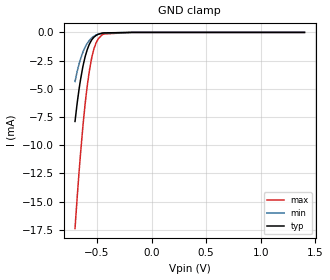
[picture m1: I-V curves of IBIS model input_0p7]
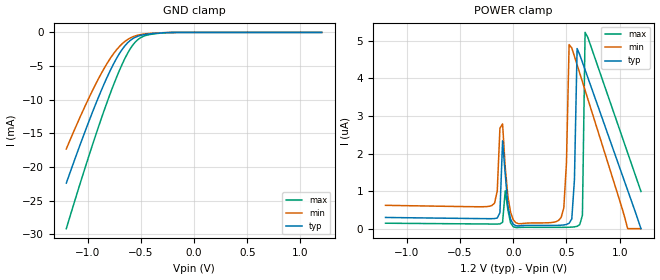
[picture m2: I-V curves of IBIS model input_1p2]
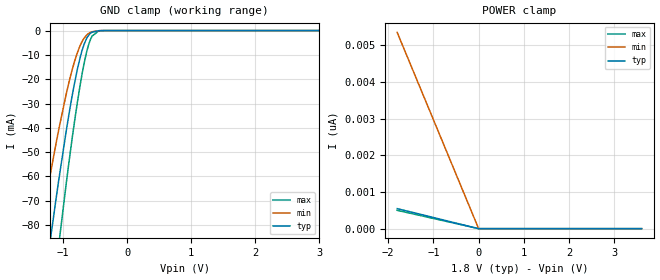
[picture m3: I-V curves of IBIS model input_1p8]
|Texas Instruments Incorporated
| 8-Bit Dual-Supply Bus Transceiver With Configurable Voltage Translation and
| 3-State Outputs
[IBIS Ver]   4.2
[File name]   sn74axc8t245.ibs
[Date]   03/06/2020
[File Rev]   1.2
[Source]
| Texas Instruments Incorporated.
| Analog-eLab Design Center, HPA
| 12500 TI Blvd
| Dallas, TX -75243
[Notes]
| Rev 1.2: 12/018/2023
| - Added input_1p2, 2p5, io_1p2 and io_2p5 model.
| Rev 1.1: 03/06/2020
| - Added input_1p8 and io_1p8 model.
| Rev 1.0: 06/08/2017
| - Initial version of the model
| - Model generated from simulations in SPECTRE
| - Model matched to SPICE simulation
| - C_comp although listed in numerical order of value are
|   obtained from varying PVT conditions. For PVT conditions for
|   each specific value refer the buffer description under
|   respective [Model]. IBIS model user is responsible for using
|   appropriate C_comp to simulate for Signal Integrity.
[Disclaimer]
| This model is designed as an aid for customers of Texas Instruments.
| TI and its licensors and suppliers make no warranties, either expressed
| or implied, with respect to this  model, including the warranties of
| merchantability or fitness for a particular purpose. The model is
| provided solely on an "as is" basis. The entire risk as to its quality
| and performance is with the customer.
[Copyright]
(C) Copyright 2017 Texas Instruments Incorporated.All rights reserved.
|   SN74AXC8T245PW
| Marketing part#   Digital Voltage Range   Package-type   #pins
| SN74AXC8T245PW   0.65V-3.6V   TSSOP   24
[Component]   SN74AXC8T245PW
[Manufacturer]  TI
[Package]   |24 TSSOP - PW package
|   typ   min   max
R_pkg   0.1143375   0.06811   0.12769
L_pkg   3.405334167nH   2.85598nH   4.17092nH
C_pkg   0.565412083pF   0.46044pF   0.71557pF
[Pin]  signal_name model_name   R_pin   L_pin   C_pin
1   VCCA   power   0.06958   3.86966nH   0.71557pF
2   DIR1   input   0.12094   3.80225nH   0.66679pF
3   A1   io   0.12769   3.54754nH   0.57242pF
4   A2   io   0.12362   3.25170nH   0.50771pF
5   A3   io   0.11601   3.02250nH   0.49462pF
6   A4   io   0.10931   2.86990nH   0.46105pF
7   A5   io   0.10845   2.85719nH   0.46044pF
8   A6   io   0.11376   2.99109nH   0.49241pF
9   A7   io   0.11998   3.20023nH   0.50408pF
10   A8   io   0.12312   3.48368nH   0.56447pF
11   DIR2   input   0.12091   3.81199nH   0.66374pF
12   GND   gnd   0.11675   4.13953nH   0.67876pF
13   GND   gnd   0.06811   3.82650nH   0.71298pF
14   B8   io   0.12091   3.81016nH   0.66711pF
15   B7   io   0.12766   3.55445nH   0.57259pF
16   B6   io   0.12359   3.25719nH   0.50787pF
17   B5   io   0.11599   3.02618nH   0.49474pF
18   B4   io   0.10929   2.87119nH   0.46118pF
19   B3   io   0.10845   2.85598nH   0.46051pF
20   B2   io   0.11377   2.98788nH   0.49236pF
21   B1   io   0.12   3.19513nH   0.50408pF
22   nOE   input   0.12314   3.47698nH   0.56494pF
23   VCCB   power   0.12375   3.84820nH   0.66804pF
24   VCCB   power   0.11932   4.17092nH   0.68143pF
|   SN74AXC8T245RHL
| Marketing part#   Digital Voltage Range   Package-type   #pins
| SN74AXC8T245RHL   0.65V-3.6V   YQFN   24
[Component]   SN74AXC8T245RHL
[Manufacturer]  TI
[Package]   |24 YQFN - RHL package
|   typ   min   max
R_pkg   0.085   0.058   0.116
L_pkg   1.593n   1.101n   2.229n
C_pkg   0.258p   0.219p   0.337p
[Pin]  signal_name model_name   R_pin   L_pin   C_pin
1   VCCA   power   0.0589   1.5334n   0.3373p
2   DIR1   input   0.1148   2.1925n   0.2676p
3   A1   io   0.0984   1.7889n   0.2917p
4   A2   io   0.0841   1.4994n   0.2570p
5   A3   io   0.0723   1.2607n   0.2333p
6   A4   io   0.0655   1.1245n   0.2200p
7   A5   io   0.0637   1.1101n   0.2185p
8   A6   io   0.0688   1.2432n   0.2289p
9   A7   io   0.0788   1.4543n   0.2506p
10   A8   io   0.0925   1.7374n   0.2753p
11   DIR2   input   0.1138   2.1938n   0.2623p
12   GND   gnd   0.1074   2.0415n   0.2530p
13   GND   gnd   0.0585   1.5096n   0.3326p
14   B8   io   0.1153   2.1253n   0.2676p
15   B7   io   0.0992   1.7605n   0.2916p
16   B6   io   0.0837   1.4781n   0.2571p
17   B5   io   0.0716   1.2733n   0.2332p
18   B4   io   0.0645   1.1262n   0.2200p
19   B3   io   0.0636   1.1010n   0.2188p
20   B2   io   0.0699   1.2254n   0.2290p
21   B1   io   0.0807   1.4310n   0.2511p
22   nOE   input   0.0943   1.7202n   0.2780p
23   VCCB   power   0.1164   2.2294n   0.2692p
24   VCCB   power   0.1093   2.0732n   0.2573p
|   SN74AXC8T245RJW
| Marketing part#   Digital Voltage Range   Package-type   #pins
| SN74AXC8T245RJW   0.65V-3.6V   uQFN   24
[Component]   SN74AXC8T245RJW
[Manufacturer]  TI
[Package]   |24 uQFN - RKT package
|   typ   min   max
R_pkg   0.078075   0.04588   0.12141
L_pkg   0.978537917nH   0.60336nH   1.54474nH
C_pkg   0.304233333pF   0.23351pF   0.36249pF
[Pin]  signal_name model_name   R_pin   L_pin   C_pin
1   DIR1   input   0.11918   1.51673nH   0.27692pF
2   A1   io   0.10353   1.29938nH   0.30726pF
3   A2   io   0.08751   1.07368nH   0.36249pF
4   A3   io   0.07203   0.86586nH   0.33880pF
5   A4   io   0.05935   0.69679nH   0.32139pF
6   A5   io   0.0523   0.60336nH   0.31235pF
7   A6   io   0.05388   0.62418nH   0.31443pF
8   A7   io   0.06332   0.74959nH   0.32669pF
9   A8   io   0.07633   0.93332nH   0.25699pF
10   DIR2   input   0.09587   1.19534nH   0.23351pF
11   GND   gnd   0.08919   1.06264nH   0.27090pF
12   GND   gnd   0.04588   0.78601nH   0.30916pF
13   B8   io   0.0958   1.19956nH   0.23938pF
14   B7   io   0.08139   1.00661nH   0.26883pF
15   B6   io   0.06751   0.81220nH   0.33269pF
16   B5   io   0.05632   0.66473nH   0.31784pF
17   B4   io   0.05189   0.60699nH   0.31231pF
18   B3   io   0.05639   0.66565nH   0.31794pF
19   B2   io   0.06763   0.81366nH   0.33284pF
20   B1   io   0.0824   1.01033nH   0.35462pF
21   nOE   input   0.09804   1.22986nH   0.28985pF
22   VCCB   power   0.12141   1.54474nH   0.26570pF
23   VCCB   power   0.1169   1.43698nH   0.29681pF
24   VCCA   power   0.05975   1.08672nH   0.34190pF
|   Model Selectors
[Model Selector] input
input_0p7   0.7V   digital Input
input_1p8   1.8V   digital Input
input_3p3   3.3V   digital Input
[Model Selector] io
io_0p7   0.7V   digital I/O
io_1p8   1.8V   digital I/O
io_3p3   3.3V   digital I/O
| Models and submodels in the file (10): input_0p7 (Input), input_1p2 (Input), input_1p8 (Input), input_2p5 (Input), input_3p3 (Input), io_0p7 (I/O), io_1p2 (I/O), io_1p8 (I/O), io_2p5 (I/O), io_3p3 (I/O)
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|   input_0p7 Model
[Model]   input_0p7
Model_type   Input
Vinl = 0.21
Vinh = 0.49
|   typ   min   max
C_comp   7.40696E-13   6.45127E-13   8.98734E-13
[Model spec]
|subparameter
Vinl   0.21   0.195   0.225
Vinh   0.49   0.455   0.525
| Where Nom  PVT is Nominal Process, 0.7V, 27C
|   Fast PVT is Strong Process,  0.75V, -40C
|   Slow PVT is Weak Process,   0.65, 130C
[Voltage Range]   0.7   0.65   0.75
|Junction Temperature
[Temperature Range]   27   130   -40
[Power Clamp Reference]   0.7   0.65   0.75
[GND Clamp Reference]   0   0   0
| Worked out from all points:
|   GND clamp passes 1 mA (typ) near -0.57 V on its own axis
[GND Clamp]
|   Voltage   I(typ)   I(min)   I(max)
-700mV    -7.896mA   -4.354mA   -17.4mA
-676.9mV  -6.033mA   -3.335mA   -14.2mA
-651.7mV  -4.329mA   -2.43mA    -11.02mA
-624.4mV  -2.873mA   -1.673mA   -7.992mA
-588.7mV  -1.545mA   -978.4uA   -4.797mA
-567.7mV  -1.026mA   -696.2uA   -3.358mA
-548.8mV  -691.6uA   -504.6uA   -2.342mA
-527.8mV  -434.7uA   -346.8uA   -1.503mA
-487.9mV  -168.3uA   -161.7uA   -574.9uA
-454.3mV  -71.1uA    -80.61uA   -230.7uA
-175mV    -4.456nA   -77.57nA   0A
1.4V      0A         0A         0A
[POWER Clamp]
|   Voltage   I(typ)   I(min)   I(max)
-700mV    0A         0A         0A
0V        0A         0A         0A
1.4V      0A         0A         0A
|   input_1p2 Model
[Model]   input_1p2
Model_type   Input
Vinl = 0.45
Vinh = 0.75
|   typ   min   max
C_comp   1.882pF   1.843pF   1.914pF
| Where Nom  PVT is Nominal Process, 1.2V,  27C
|   Fast PVT is Strong Process,  1.08V, -40C
|   Slow PVT is Weak Process,   1.32V, 130C
[Voltage Range]   1.2   1.08   1.32
|Junction Temperature
[Temperature Range]   27   125   -40
[Power Clamp Reference]   1.2   1.08   1.32
[GND Clamp Reference]   0   0   0
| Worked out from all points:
|   GND clamp passes 1 mA (typ) near -0.58 V on its own axis
[GND Clamp]
|   Voltage   I(typ)   I(min)   I(max)
-1.2V     -22.38mA   -17.31mA   -29.14mA
-1.075V   -16.88mA   -12.73mA   -22.69mA
-950mV    -11.68mA   -8.497mA   -16.5mA
-850mV    -7.838mA   -5.493mA   -11.83mA
-775mV    -5.268mA   -3.579mA   -8.565mA
-700mV    -3.113mA   -2.076mA   -5.605mA
-625mV    -1.561mA   -1.066mA   -3.12mA
-575mV    -920.5uA   -654.6uA   -1.868mA
-525mV    -552uA     -401.8uA   -1.034mA
-425mV    -234.6uA   -164uA     -348.1uA
-225mV    -22.14uA   -17.06uA   -25.5uA
1.2V      0A         0A         0A
[POWER Clamp]
|   Voltage   I(typ)   I(min)   I(max)
-1.2V     298.2nA    621.6nA    145.1nA
-200mV    266.1nA    616nA      123.4nA
-100mV    2.341uA    2.79uA     168.8nA
0V        118.3nA    238.2nA    51.34nA
425mV     88.99nA    217.6nA    34.54nA
475mV     98.89nA    549.3nA    35.51nA
525mV     144.1nA    4.902uA    38.32nA
575mV     1.304uA    4.589uA    48.09nA
600mV     4.796uA    4.364uA    62.93nA
650mV     4.431uA    3.912uA    359.3nA
675mV     4.23uA     3.686uA    5.227uA
1.2V      0A         0A         989.8nA
|   input_1p8 Model
[Model]   input_1p8
Model_type   Input
Vinl = 0.7
Vinh = 1.6
|   typ   min   max
C_comp   1.392pf   0.843pf   1.994pF
| Where Nom  PVT is Nominal Process, 1.8V,  27C
|   Fast PVT is Strong Process,  1.98V, -40C
|   Slow PVT is Weak Process,   1.62V, 130C
[Voltage Range]   1.8   1.62   1.98
|Junction Temperature
[Temperature Range]   27   130   -40
[Power Clamp Reference]   1.8   1.62   1.98
[GND Clamp Reference]   0   0   0
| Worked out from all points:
|   GND clamp passes 1 mA (typ) near -0.56 V on its own axis
[GND Clamp]
|   Voltage   I(typ)   I(min)   I(max)
-1.8V     -210.9mA   -157.9mA   -261.6mA
-1.319V   -109.8mA   -77.26mA   -146mA
-1.206V   -87.46mA   -60.12mA   -119.6mA
-1.12V    -71.04mA   -47.78mA   -99.81mA
-1.066V   -61.14mA   -40.45mA   -87.72mA
-952.2mV  -41.52mA   -26.26mA   -63.25mA
-903.6mV  -33.72mA   -20.8mA    -53.27mA
-779.4mV  -16.26mA   -9.28mA    -30.01mA
-676.8mV  -6.025mA   -3.331mA   -14.19mA
-579.6mV  -1.299mA   -846.1uA   -4.132mA
-385.2mV  -10.15uA   -16.94uA   -26.09uA
3.6V      0A         0A         0A
[POWER Clamp]
|   Voltage   I(typ)   I(min)   I(max)
-1.8V     546.7pA    5.348nA    499.5pA
0V        0A         0A         0A
3.6V      0A         0A         0A
